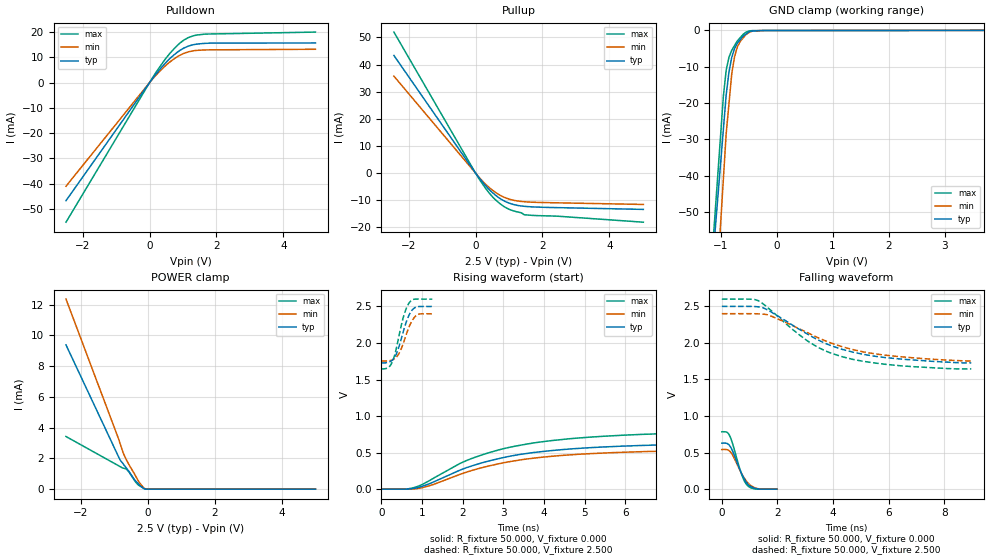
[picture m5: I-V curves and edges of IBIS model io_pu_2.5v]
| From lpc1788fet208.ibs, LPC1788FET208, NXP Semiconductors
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[Model]   io_pu_2.5v
Model_type I/O
Vinl=7.500E-01
Vinh=1.750E+00
Vref=0.000E+00
Rref=1.000E+06
Cref=0.000E+00
Vmeas=1.250E+00
C_comp   6.060E-13   5.760E-13   6.360E-13
[Voltage Range]   2.500E+00   2.400E+00   2.600E+00
[POWER Clamp Reference]   2.500E+00   2.400E+00   2.600E+00
[GND Clamp Reference]   0.000E+00   0.000E+00   0.000E+00
[Pullup Reference]   2.500E+00   2.400E+00   2.600E+00
[Pulldown Reference]   0.000E+00   0.000E+00   0.000E+00
[Temperature Range]   25   85   -40
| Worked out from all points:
|   slope of the pulldown table from 0 to 0.375 V, typ, clamps not added: 60.1 ohm
|   slope of the pullup table from 0 to 0.375 V, typ, clamps not added: 66.3 ohm
|   GND clamp passes 1 mA (typ) near -0.55 V on its own axis
|   POWER clamp passes 1 mA (typ) near -0.52 V on its own axis
|   rising waveform, R_fixture 50.000, V_fixture 0.000: 20-80 % time 2.39ns typ, 2.4ns min, 2.39ns max; typ from 0 V to 0.629 V
|   falling waveform, R_fixture 50.000, V_fixture 0.000: 20-80 % time 421ps typ, 454ps min, 375ps max; typ from 0.629 V to 0 V
|   rising waveform, R_fixture 50.000, V_fixture 2.500: 20-80 % time 260ps typ, 267ps min, 245ps max; typ from 1.73 V to 2.5 V
|   falling waveform, R_fixture 50.000, V_fixture 2.500: 20-80 % time 2.52ns typ, 2.66ns min, 2.25ns max; typ from 2.5 V to 1.73 V
[GND Clamp]
-2.5V     -320.9mA   -428.2mA   -355.8mA
-950mV    -27.31mA   -41.03mA   -18.18mA
-900mV    -17.84mA   -28.54mA   -11.01mA
-850mV    -11.49mA   -20.22mA   -7.415mA
-800mV    -7.413mA   -11.9mA    -5.476mA
-750mV    -5.014mA   -7.253mA   -4.181mA
-700mV    -3.535mA   -4.543mA   -2.887mA
-650mV    -2.594mA   -3.07mA    -2.015mA
-550mV    -1.057mA   -1.212mA   -539.5uA
-400mV    -147.5uA   -112.4uA   -63.11uA
-200mV    -36.9uA    -30.37uA   -38.72uA
5V        16.89uA    16.03uA    16.38uA
[Power Clamp]
-2.44V    9.388mA    12.37mA    3.427mA
-864.3mV  2.069mA    3.227mA    1.515mA
-824.4mV  1.888mA    2.953mA    1.468mA
-704.7mV  1.555mA    2.207mA    1.357mA
-644.9mV  1.391mA    1.935mA    1.317mA
-565.1mV  1.161mA    1.609mA    1.121mA
-405.5mV  639.5uA    1.023mA    599.2uA
-285.8mV  358.5uA    551.8uA    272.7uA
-206mV    179.2uA    299.1uA    176uA
-106.3mV  38.2uA     67.27uA    36.76uA
-46.45mV  0A         0A         0A
5V        0A         0A         0A
[Pullup]
-2.44V    43.36mA    35.74mA    51.99mA
73.23mV   -1.212mA   -1.083mA   -1.512mA
412.3mV   -6.134mA   -5.372mA   -7.408mA
571.9mV   -7.907mA   -6.919mA   -9.588mA
731.5mV   -9.384mA   -8.178mA   -11.31mA
891mV     -10.51mA   -9.115mA   -12.66mA
1.071V    -11.38mA   -9.854mA   -13.7mA
1.37V     -12.17mA   -10.49mA   -14.71mA
1.47V     -12.3mA    -10.6mA    -15.43mA
2.447V    -12.77mA   -11mA      -15.93mA
5.02V     -13.43mA   -11.6mA    -18.15mA
[Pulldown]
-2.5V     -46.78mA   -41.06mA   -55.31mA
133mV     2.372mA    2.061mA    2.84mA
571.8mV   9.068mA    7.781mA    11mA
910.9mV   12.75mA    10.83mA    15.67mA
1.21V     14.64mA    12.31mA    18.05mA
1.409V    15.21mA    12.73mA    18.81mA
1.629V    15.5mA     12.89mA    19.14mA
4.96V     15.67mA    13.17mA    19.98mA
[Rising Waveform]
R_fixture = 50.000
V_fixture = 0.000
V_fixture_min = 0.000
V_fixture_max = 0.000
|  time   V(typ)   V(min)   V(max)
0s        0V         0V         0V
589.4ps   280.9uV    -130uV     680.1uV
819.1ps   13.11mV    3.684mV    24.01mV
1.169ns   71.91mV    44.1mV     113.2mV
1.938ns   262mV      203.9mV    353.7mV
2.228ns   319mV      256.6mV    421.4mV
2.937ns   424.8mV    353.1mV    545.1mV
3.736ns   500.7mV    423.6mV    631.9mV
5.984ns   589.9mV    505.2mV    739.5mV
9.53ns    629.3mV    541.7mV    784.8mV
[Falling Waveform]
R_fixture = 50.000
V_fixture = 0.000
V_fixture_min = 0.000
V_fixture_max = 0.000
|  time   V(typ)   V(min)   V(max)
0s        629.3mV    541.7mV    784.8mV
179.1ps   625.7mV    540.3mV    778.6mV
288.6ps   591.3mV    517.2mV    725.2mV
410ps     499.6mV    450.4mV    593.4mV
706.5ps   215.8mV    216.6mV    208.4mV
815.9ps   132.4mV    146.7mV    107.5mV
915.4ps   76.07mV    94.62mV    51.88mV
1.05ns    32.54mV    47.11mV    17.48mV
1.284ns   3.901mV    7.986mV    310.5uV
1.98ns    0V         0V         0V
[Rising Waveform]
R_fixture = 50.000
V_fixture = 2.500
V_fixture_min = 2.400
V_fixture_max = 2.600
|  time   V(typ)   V(min)   V(max)
0s        1.727V     1.754V     1.644V
168.7ps   1.735V     1.755V     1.665V
267.9ps   1.766V     1.768V     1.742V
347.2ps   1.827V     1.796V     1.882V
436.5ps   1.959V     1.863V     2.112V
550ps     2.181V     2.015V     2.375V
684.6ps   2.389V     2.227V     2.552V
773.9ps   2.462V     2.324V     2.594V
880ps     2.495V     2.385V     2.601V
1.25ns    2.5V       2.4V       2.6V
[Falling Waveform]
R_fixture = 50.000
V_fixture = 2.500
V_fixture_min = 2.400
V_fixture_max = 2.600
|  time   V(typ)   V(min)   V(max)
0s        2.5V       2.4V       2.6V
998.9ps   2.5V       2.4V       2.599V
1.299ns   2.494V     2.398V     2.58V
1.788ns   2.42V      2.365V     2.438V
3.087ns   2.119V     2.14V      2.026V
3.676ns   2.002V     2.036V     1.9V
4.275ns   1.918V     1.954V     1.817V
5.104ns   1.843V     1.876V     1.748V
5.913ns   1.798V     1.831V     1.706V
8.97ns    1.727V     1.754V     1.644V
[Ramp]
dV/dt_r   3.7967E-01/2.3879E-09   3.2490E-01/2.3920E-09   4.7355E-01/2.3872E-09
dV/dt_f   4.6402E-01/2.5227E-09   3.8788E-01/2.6605E-09   5.7347E-01/2.2506E-09
R_load = 50
